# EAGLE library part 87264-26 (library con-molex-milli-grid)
RECEPTACAL
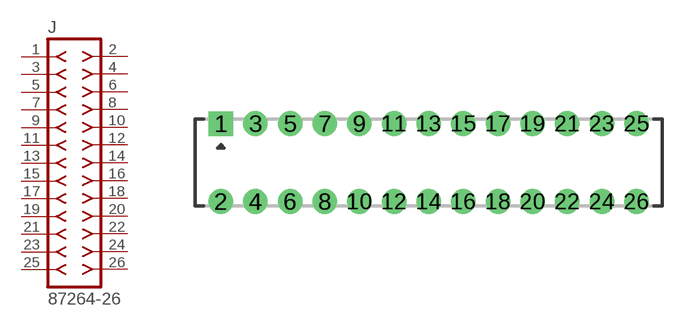
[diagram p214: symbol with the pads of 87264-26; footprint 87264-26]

Designator prefix J

## 87264-26  [87264-26]
1  1  pas
2  2  pas
3  3  pas
4  4  pas
5  5  pas
6  6  pas
7  7  pas
8  8  pas
9  9  pas
10  10  pas
11  11  pas
12  12  pas
13  13  pas
14  14  pas
15  15  pas
16  16  pas
17  17  pas
18  18  pas
19  19  pas
20  20  pas
21  21  pas
22  22  pas
23  23  pas
24  24  pas
25  25  pas
26  26  pas

## Footprint 87264-26 (pad centres in mm)
RECEPTACAL Dual Row, Side Entry
drill 0.914 square: 1 -12,2.25
drill 0.914: 2 -12,-2.25; 3 -10,2.25; 4 -10,-2.25; 5 -8,2.25; 6 -8,-2.25; 7 -6,2.25; 8 -6,-2.25; 9 -4,2.25; 10 -4,-2.25; 11 -2,2.25; 12 -2,-2.25; 13 0,2.25; 14 0,-2.25; 15 2,2.25; 16 2,-2.25; 17 4,2.25; 18 4,-2.25; 19 6,2.25; 20 6,-2.25; 21 8,2.25; 22 8,-2.25; 23 10,2.25; 24 10,-2.25; 25 12,2.25; 26 12,-2.25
